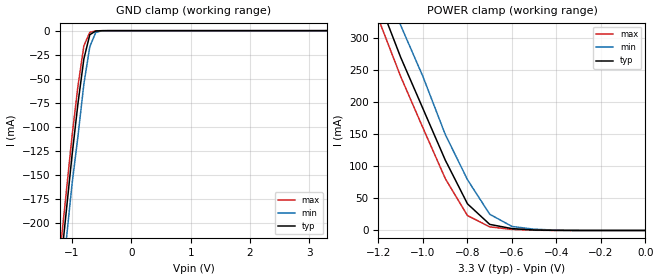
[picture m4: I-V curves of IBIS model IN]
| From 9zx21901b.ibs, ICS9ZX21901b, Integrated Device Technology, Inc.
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|   Model IN
[Model]   IN
Model_type   Input
Polarity   Inverting
Enable   Active-High
Vinl =   1.00V
Vinh =   2.00V
C_comp   3.40pF   2.85pF   3.95pF
[Temperature Range]   27.00   70.00   0.000
[Voltage Range]   3.30V   3.00V   3.60V
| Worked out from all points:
|   GND clamp passes 1 mA (typ) near -0.62 V on its own axis
|   POWER clamp passes 1 mA (typ) near -0.51 V on its own axis
[GND_clamp]
| voltage   I(typ)   I(min)   I(max)
-3.3V     -1.54A     -1.54A     -1.54A
-1.2V     -250mA     -270mA     -230mA
-1.1V     -190mA     -220mA     -170mA
-1V       -130mA     -160mA     -110mA
-900mV    -75.97mA   -110mA     -57.72mA
-800mV    -29.3mA    -55.39mA   -15.7mA
-700mV    -4.2mA     -16.67mA   -1.77mA
-600mV    -420uA     -1.81mA    -210uA
-500mV    -36.28uA   -150uA     -14.74uA
3.3V      150pA      92.22uA    -1.21nA
[POWER_clamp]
| voltage   I(typ)   I(min)   I(max)
-3.3V     2.31A      2.35A      2.29A
-1.2V     360mA      410mA      330mA
-1.1V     270mA      320mA      240mA
-1V       190mA      240mA      160mA
-900mV    110mA      150mA      81.19mA
-800mV    41.59mA    79.25mA    23.27mA
-700mV    9.51mA     25.32mA    5.62mA
-600mV    2.91mA     6.31mA     1.67mA
-500mV    750uA      1.96mA     350uA
-300mV    20.87uA    92.22uA    6.56uA
0V        150pA      200pA      160pA
